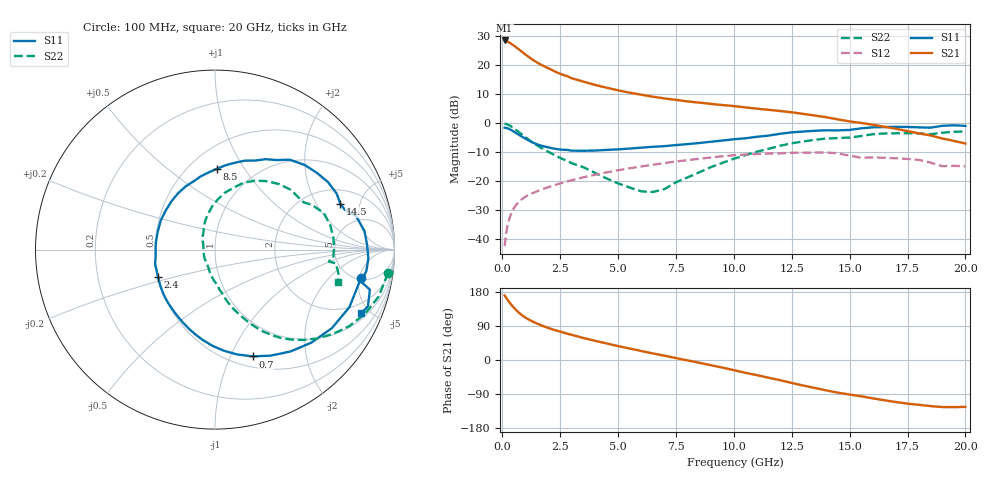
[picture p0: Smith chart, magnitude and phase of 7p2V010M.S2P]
! Infineon Technologies  Discrete & RF Semiconductors
! bfp620
! VCE =  2.0 V,  IC =  10 mA
! Common Emitter S-Parameters:  Sep 2002
# GHz  S  MA  R  50
!  f  S11  S21  S12  S22
! GHz  MAG  ANG  MAG  ANG  MAG  ANG  MAG  ANG
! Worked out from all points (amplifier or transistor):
!   59 points, 100 MHz to 20 GHz, reference 50 ohm
!   highest |S21| = 28.3 dB at 100 MHz (marker M1)
!   |S21| within 3 dB of that: start of sweep to 702.3 MHz
!   unconditionally stable (mu >= 1): 4.015 GHz to 10.71 GHz; 17.11 GHz to end of sweep
!   at 1 GHz: K = 0.50, MSG = 24.5 dB, |S12| = -25.4 dB
!   at 5.5 GHz: K = 1.05, MAG = 11.7 dB, |S12| = -15.6 dB
!   at 20 GHz: K = 1.32, MAG = 0.5 dB, |S12| = -14.9 dB
!   S11 on the Smith chart (normalised r, x): 100 MHz: 5.14, -5.27; 700 MHz: 0.62, -1.22; 2.4 GHz: 0.50, -0.17; 8.5 GHz: 0.67, +0.76; 14.5 GHz: 2.88, +3.27; 20 GHz: 1.31, -4.44
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0.1  0.8283 -11.2  26.14 170.5  0.0076 78.2  0.9722 -7.7
0.2  0.8146 -23.2  25.31 161.1  0.0154 75.8  0.9489 -16.0
0.3  0.7846 -33.9  24.11 152.7  0.0224 71.7  0.9091 -23.2
0.4  0.7467 -43.9  22.73 145.1  0.0286 67.8  0.8601 -29.8
0.5  0.7067 -53.4  21.29 138.1  0.0342 64.2  0.8075 -35.6
0.6  0.6678 -62.2  19.88 131.6  0.0391 61.1  0.7546 -41.0
0.7  0.6312 -70.5  18.53 125.8  0.0434 58.4  0.7034 -45.7
0.8  0.597 -78.1  17.27 120.6  0.0473 56.1  0.655 -49.9
1  0.5358 -91.6  14.99 111.9  0.0537 52.5  0.5682 -56.7
1.3  0.4628 -108.6  12.28 101.9  0.0618 48.9  0.4645 -63.9
1.5  0.4284 -118.4  10.94 96.3  0.0667 47.4  0.4115 -67.6
1.8  0.3948 -131.7  9.436 88.8  0.074 45.6  0.3503 -72.3
2.4  0.3524 -154.2  7.246 76.7  0.0885 42.5  0.2618 -79.4
3.5  0.332 174.2  5.129 58.1  0.1161 35.9  0.1733 -91.8
5  0.3507 141.3  3.633 36.7  0.1535 25.1  0.0913 -118.9
7  0.3983 107.5  2.636 11.5  0.2037 8.7  0.0725 154.4
8.5  0.4507 88.7  2.231 -7.2  0.2416 -5.4  0.141 116.5
10.5  0.5443 65.7  1.847 -33.8  0.2855 -27.8  0.2787 87.1
13.5  0.7332 30.9  1.336 -73.8  0.3085 -61.6  0.5114 45.4
14.5  0.7436 20.0  1.148 -86.3  0.2993 -76.4  0.5476 32.2
17  0.8559 -3.3  0.793 -111.0  0.2462 -92.7  0.6628 5.9
20  0.8892 -23.5  0.442 -123.8  0.1792 -104.3  0.7091 -14.8
